FUNCTION_BLOCK FB94
TITLE =Get Fault State
//*****************************************************************************
//* maxon motor ag
//* R&D
//* all rights reserved
//*****************************************************************************
//* Summary:  Read device status
//*
//* Remarks:
//*
//* Created under: STEP7 REV5.2+SP1
//*****************************************************************************
//* History:
//* 19.05.2004 | INA   first release
//*
//*
//*****************************************************************************
//

AUTHOR:INA
FAMILY:StateMac
NAME:GetFauSt
VERSION:00.01


VAR_INPUT

Read : BOOL //A rising edge start the command

  NodeID : BYTE //Adress of the maxon device

END_VAR
VAR_OUTPUT
  Done : BOOL //Data valid flag is TRUE if data were available

  Err : BOOL //Error flag is TRUE if an Error has occured, see ErrNo for more details

  ErrNo : DINT //Contains detailed error information

  IsInErrorState : BOOL //Device fault state

END_VAR
VAR
  xEdgeMerker : BOOL //Edge Merker

  xEdgeFlag : BOOL //Edge Flag

  xStep : INT
  xStatusword : WORD
  xFault : WORD  := W#16#8
  xFaultReactionActive : WORD  := W#16#F
END_VAR

BEGIN

NETWORK
TITLE = Activate the service function
//

// SDO Read "Get Fault State"

       U    #Read
       FP   #xEdgeFlag                   // recognize a positiv edge of the Read signal
       =    #xEdgeMerker                 // and set the xEdgeMerker for one cycle to true

       L    #xStep
       L    0
       ==I
       U    #xEdgeMerker
       SPB  nstp                         // iStep = 1 -> fnc1

       L    #xStep                       // jump list
       SPL  List
       SPA  rdef
       SPA  fnc1
       SPA  fncE
List  :SPA  rdef

rdef  :NOP  0
       R    #Done                        // reset Done
       R    #Err                         // reset Error
       L    0
       T    #xStep                       // iStep = 0
       SPA  end

fnc1  :NOP  0
       CALL FC1
         NodeID:=#NodeID
         Index:=DW#16#00006041
         SubIndex:=DW#16#00000000
         RET_VAL:=#Done
         Err:=#Err
         ErrNo:=#ErrNo

       L    DB219.DBW10
       UW   W#16#007F
       T    #xStatusword

       L    #xStatusword
       L    #xFault
       ==I
       SPB  tdis

       L    #xStatusword
       L    #xFaultReactionActive
       ==I
       SPB  tdis
       SPA  fdis

tdis  :NOP  0
       S    #IsInErrorState              // set IsEnabled
       SPA  fncE

fdis  :NOP  0
       R    #IsInErrorState              // reset IsEnabled

fncE  :NOP  0
       L    0
       T    #xStep
       SPA  end

nstp  :NOP  0
       L    #xStep
       INC            1
       T    #xStep

end   :NOP  0
END_FUNCTION_BLOCK
